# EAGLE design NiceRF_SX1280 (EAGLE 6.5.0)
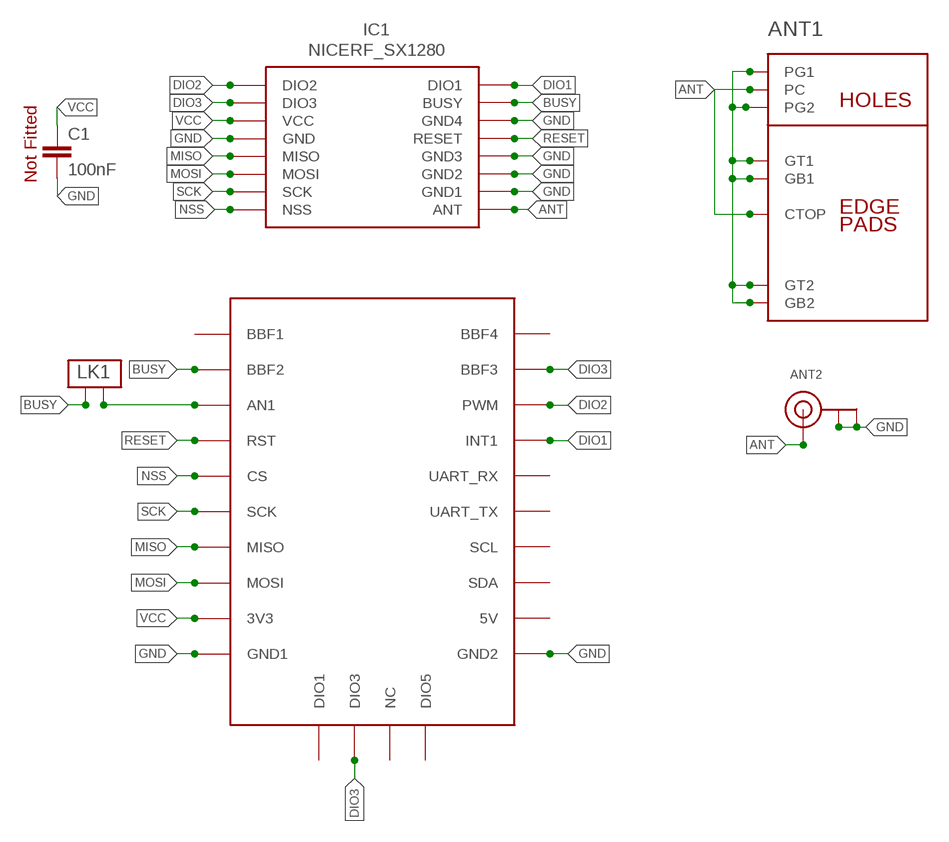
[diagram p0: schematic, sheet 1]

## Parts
ANT1  CUSTOMSMA  [CUSTOMSMA]
ANT2  ANTENNA_U.FL  [U.FL]
C1  100nF  C-EUC0805  [C0805]
IC1  NICERF_SX1280  [NICERF_SX1280]
LK1  PCB_LINK  [PCB_LINK]
U$1  BBFRIENDLY3  [PCB_SOCKET_BBFRIENDLY3]

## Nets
ANT: ANT1.CTOP ANT1.PC ANT2.3(SIGNAL) IC1.P$9(ANT)
BUSY: IC1.P$15(BUSY) LK1.P$2 U$1.BBF2
DIO1: IC1.P$16(DIO1) U$1.INT(INT1)
DIO2: IC1.P$1(DIO2) U$1.PWM
DIO3: IC1.P$2(DIO3) U$1.BBF3 U$1.DIO3
GND [VDD]: ANT1.G1 ANT1.G2 ANT1.GB1 ANT1.GB2 ANT1.GT1 ANT1.GT2 ANT2.1(GND) ANT2.2(GND) C1.2 IC1.P$4(GND) IC1.P$10(GND1) IC1.P$11(GND2) IC1.P$12(GND3) IC1.P$14(GND4) U$1.GND1 U$1.GND2
MISO: IC1.P$5(MISO) U$1.MISO
MOSI: IC1.P$6(MOSI) U$1.MOSI
N$3: LK1.P$1 U$1.AN1
NSS: IC1.P$8(NSS) U$1.CS
RESET: IC1.P$13(RESET) U$1.RST
SCK: IC1.P$7(SCK) U$1.SCK
VCC [VDD]: C1.1 IC1.P$3(VCC) U$1.3V3
Unconnected: U$1.5V U$1.BBF1 U$1.BBF4 U$1.DIO1 U$1.DIO5 U$1.NC U$1.RX(UART_RX) U$1.SCL U$1.SDA U$1.TX(UART_TX)

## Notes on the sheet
- Not Fitted

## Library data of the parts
ANT1 = con-coax:CUSTOMSMA
ANT2 = adafruit:ANTENNA_U.FL: U.FL Antenna Connector
C1 = resistor:C-EU: CAPACITOR, European symbol
IC1 = LMA2:NICERF_SX1280
LK1 = LMA2:PCB_LINK
U$1 = My_Mikrobus:BBFRIENDLY3

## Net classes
0 default: width 0.203 mm
1 POWER: width 0.635 mm
2 VDD: width 0.635 mm

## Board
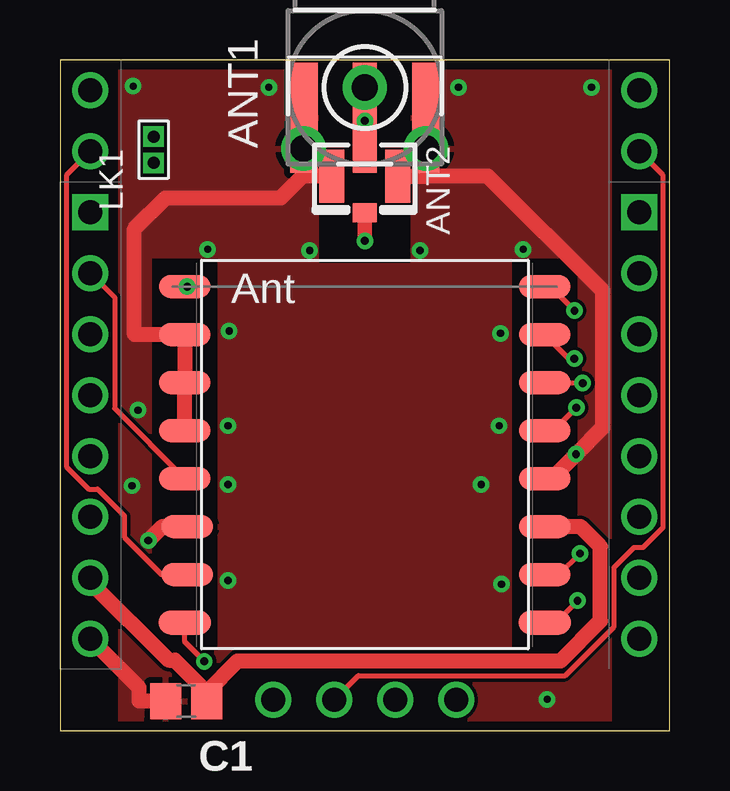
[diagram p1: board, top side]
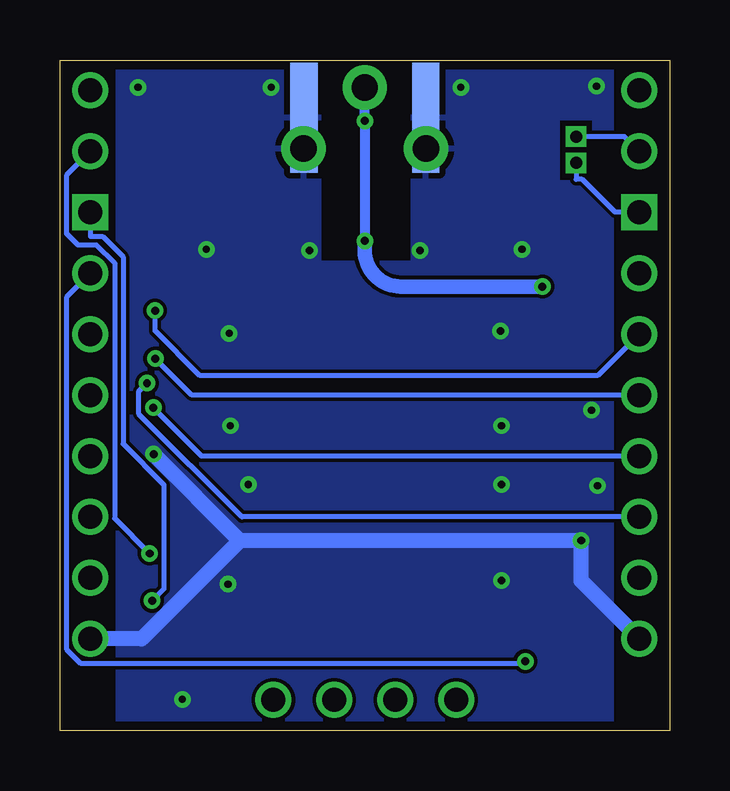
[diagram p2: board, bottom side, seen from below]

Size 25.4 x 27.94 mm. Coordinates in mm from the lower left corner, seen from the top.
Outline: 0,0 25.4,0 25.4,27.94 0,27.94 0,0
Copper layers (1*16): Top 0.0356mm / dielectric 1.5011mm / Bottom 0.0356mm
Design rules "LaenPCBOrder *": minimum track width 6mil, minimum drill 13mil, track to track 6mil, track to pad 6mil, pad to pad 6mil, via to via 6mil, smd to smd 6mil, copper to edge 15mil, drill to drill 6mil, minimum pad ring 7mil, minimum via ring 7mil, stop-mask expansion 4mil, vias tented up to drill 0mil, thermal gap 10mil
tRestrict: area 10.8,19.5 to 14.6,27.9; area 0.1,0 to 2.4,28; area 23,0 to 25.3,28; area 3.2,22.9 to 4.5,25.4; area 3.9,3.4 to 6.5,19.6; area 18.9,3.4 to 21.6,19.6
bRestrict: area 10.8,19.6 to 14.5,27.9; area 0,0 to 2.3,27.9; area 23.1,0 to 25.4,27.9; area 3.2,22.9 to 4.5,25.4

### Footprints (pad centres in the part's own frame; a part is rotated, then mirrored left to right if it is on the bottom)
CUSTOMSMA = smd 4.572 x 1.016: CTOP -1.27,0 | drill 1.1 pad 1.85: G1 -2.55,2.55; G2 -2.55,-2.55; PC 0,0 | smd 4.572 x 1.143 bottom: GB1 -1.27,2.54; GB2 -1.27,-2.54 | smd 4.572 x 1.143: GT1 -1.27,2.54; GT2 -1.27,-2.54
U.FL = smd 2.2 x 1.05: 1 0,1.375; 2 0,-1.375 | smd 0.8 x 1: 3 1.525,0
C0805 = smd 1.3 x 1.5: 1 -0.85,0; 2 0.85,0
NICERF_SX1280 = smd 2.2 x 1: P$1 -7.5,7.5; P$16 7.5,7.5 | smd 2.159 x 0.965: P$2 -7.5,5.5; P$3 -7.5,3.5; P$4 -7.5,1.5; P$5 -7.5,-0.5; P$6 -7.5,-2.5; P$7 -7.5,-4.5; P$8 -7.5,-6.5; P$9 7.5,-6.5; P$10 7.5,-4.5; P$11 7.5,-2.5; P$12 7.5,-0.5; P$13 7.5,1.5; P$14 7.4,3.5; P$15 7.4,5.5
PCB_LINK = drill 0.5 pad 0.813 square: P$1 -0.55,0; P$2 0.55,0
PCB_SOCKET_BBFRIENDLY3 = drill 1: 3V3 -11.43,3.81; 5V 11.43,3.81; BBF1 -11.43,24.13; BBF2 -11.43,21.59; BBF3 11.43,21.59; BBF4 11.43,24.13; CS -11.43,13.97; DIO1 -3.81,-1.27; DIO3 -1.27,-1.27; DIO5 3.81,-1.27; GND1 -11.43,1.27; GND2 11.43,1.27; INT 11.43,16.51; MISO -11.43,8.89; MOSI -11.43,6.35; NC 1.27,-1.27; RST -11.43,16.51; RX 11.43,13.97; SCK -11.43,11.43; SCL 11.43,8.89; SDA 11.43,6.35; TX 11.43,11.43 | drill 1 square: AN1 -11.43,19.05; PWM 11.43,19.05

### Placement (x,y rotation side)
ANT1  12.7,26.8 90 top
ANT2  12.7,23.1 270 top
C1  5.26,1.23 180 top
IC1  12.7,12 180 top
LK1  3.9,24.2 90 top
U$1  12.7,2.55 0 top

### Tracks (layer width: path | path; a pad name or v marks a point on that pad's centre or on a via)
ANT  (via drill 0.33 pad 0.69)
  Top 0.203: ANT1.PC ANT1.CTOP
  Top 0.406: ANT1.CTOP v12.7,25.4
  Top 0.61: IC1.P$9 v5.3,18.5 | v12.7,20.4 ANT2.3
  Bottom 0.406: v12.7,25.4 12.7,25.35 | 12.7,25.35 v12.7,20.4 | 12.7,25.35 ANT1.PC
  Bottom 0.61: v5.3,18.5 10.6,18.5 11.2,18.5 arc90 12.7,20 v12.7,20.4
BUSY
  Top 0.203: U$1.BBF2 0.26,23.13 0.26,10.99 1.2,10.06 1.57,10.06 2.68,8.95 2.68,8.06 4.24,6.5 IC1.P$15
  Bottom 0.203: U$1.BBF2 1.88,24.75 LK1.P$2
DIO1  (via drill 0.33 pad 0.69)
  Top 0.203: v6.01,2.88 5.2,3.69 IC1.P$16
  Bottom 0.203: U$1.INT 25.14,18.05 25.14,3.39 24.55,2.81 6.08,2.81 v6.01,2.88
DIO2  (via drill 0.33 pad 0.69)
  Top 0.203: v21.56,5.41 20.65,4.5 IC1.P$1
  Bottom 0.203: U$1.PWM 24.13,20.6 23.63,20.6 22.77,19.74 22.77,11.94 21.07,10.24 21.07,5.91 v21.56,5.41
DIO3  (via drill 0.33 pad 0.69)
  Top 0.203: v21.67,7.38 20.79,6.5 IC1.P$2 | U$1.DIO3 12.43,2.28 21.05,2.28 23.09,4.33 23.09,6.8 23.92,7.63 24.3,7.63 25.13,8.46 25.13,23.14 U$1.BBF3
  Bottom 0.203: U$1.BBF3 25.13,23.14 25.13,20.72 24.65,20.24 23.88,20.24 23.13,19.48 23.13,8.84 v21.67,7.38
GND  (via drill 0.3 pad 0.69, 0.33 pad 0.69)
  Top 0.635: 15.25,23.1 17.83,23.1 22.62,18.32 22.62,12.63 v21.5,11.52 20.48,10.5 IC1.P$4 | C1.2 3.29,1.23 3.29,1.8 U$1.GND1 | ANT2.2 10.15,23.1 | 10.15,23.1 ANT1.G1 ANT1.GB1 | ANT2.1 15.25,23.1 | IC1.P$12 IC1.P$11 IC1.P$10 4.99,16.5 3.1,16.5 3.1,20.9 4.4,22.2 9.2,22.2 10.1,23.1 10.15,23.1 | IC1.P$14 4.27,8.5 v3.69,7.92 | 15.25,23.1 ANT1.G2 ANT1.GB2
  Bottom 0.635: ANT1.G2 ANT1.GB2 | ANT1.G1 ANT1.GB1 | 17.9,7.92 22,3.82 U$1.GND2 | 17.9,7.92 v21.5,11.52 | 17.9,7.92 v3.69,7.92 3.69,6.24 U$1.GND1 | 17.9,7.92
  other vias: 3.25,13.35 3,10.2 6.15,20.05 19.3,20.05 10.4,20 15,20 7,12.7 7,10.25 7,6.25 18.4,6.1 17.55,10.25 18.3,12.7 7.05,16.65 18.35,16.55 3.05,26.85 8.7,26.8 16.6,26.8 22.15,26.8 20.3,1.3
  pour Top: 0,27.9 25.4,27.9 25.4,0 0,0
  pour Bottom: 0,27.9 25.4,27.9 25.4,0 0,0
MISO  (via drill 0.33 pad 0.69)
  Top 0.203: v21.51,13.45 20.56,12.5 IC1.P$5
  Bottom 0.203: U$1.MISO 19.5,11.44 v21.51,13.45
MOSI  (via drill 0.33 pad 0.69)
  Top 0.203: v21.78,14.48 20.22,14.48 IC1.P$6
  Bottom 0.203: U$1.MOSI 17.82,8.9 22.11,13.19 22.11,14.14 v21.78,14.48
N$3
  Bottom 0.203: LK1.P$1 3.9,22.97 3.64,22.97 2.27,21.6 U$1.AN1
NSS  (via drill 0.33 pad 0.69)
  Top 0.203: v21.44,17.5 20.44,18.5 IC1.P$8
  Bottom 0.203: U$1.CS 3,14.79 19.58,14.79 21.44,16.66 v21.44,17.5
RESET
  Top 0.203: U$1.RST 2.27,18.06 2.27,13.43 IC1.P$13
SCK  (via drill 0.33 pad 0.69)
  Top 0.203: IC1.P$7 21.2,15.5 v21.43,15.5 | v21.43,15.5
  Bottom 0.203: U$1.SCK 19.91,13.98 v21.43,15.5
VCC
  Top 0.635: 6.11,1.61 7.41,2.9 20.86,2.9 22.52,4.57 22.52,7.67 21.69,8.5 IC1.P$3 | U$1.3V3 1.27,6.19 4.53,2.93 4.79,2.93 6.11,1.61 | 6.11,1.61 C1.1

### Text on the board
Notes: 220219 | LK1 | NiceRF_SX1280 | ANT | 16 | 1 | C1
